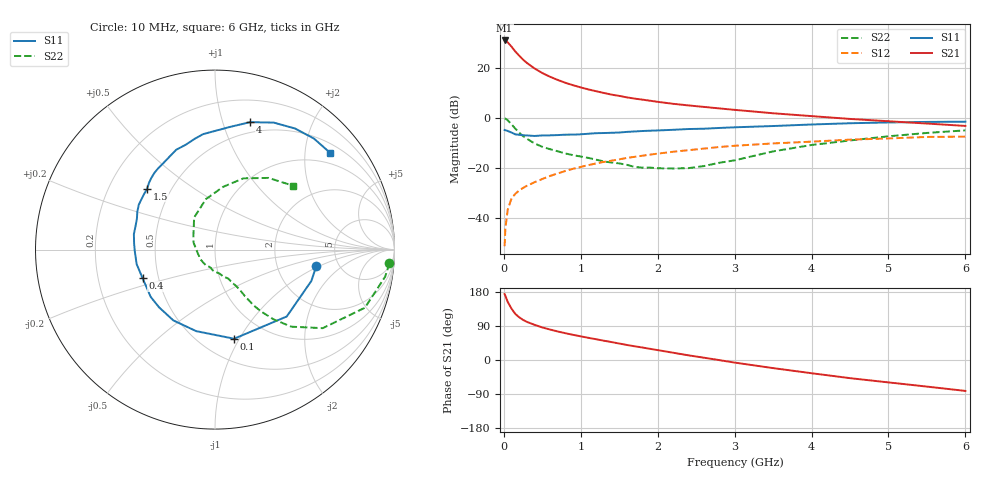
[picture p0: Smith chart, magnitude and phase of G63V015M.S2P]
! SIEMENS Small Signal Semiconductors
! BFG193
! Si NPN RF Bipolar Junction Transistor in SOT223
! VCE = 3 V  IC = 15 mA
! Common Emitter S-Parameters:  August  1996
# GHz  S  MA  R  50
!  f  S11  S21  S12  S22
! GHz  MAG  ANG  MAG  ANG  MAG  ANG  MAG  ANG
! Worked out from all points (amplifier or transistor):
!   36 points, 10 MHz to 6 GHz, reference 50 ohm
!   highest |S21| = 31.0 dB at 10 MHz (marker M1)
!   |S21| within 3 dB of that: start of sweep to 113.4 MHz
!   unconditionally stable (mu >= 1): 762.2 MHz to 2.618 GHz
!   at 250 MHz: K = 0.66, MSG = 25.7 dB, |S12| = -28.1 dB
!   at 1.4 GHz: K = 1.06, MAG = 11.7 dB, |S12| = -17.1 dB
!   at 6 GHz: K = 0.89, MSG = 2.1 dB, |S12| = -7.5 dB
!   S11 on the Smith chart (normalised r, x): 10 MHz: 3.40, -0.92; 100 MHz: 0.71, -0.95; 400 MHz: 0.41, -0.16; 1.5 GHz: 0.37, +0.34; 4 GHz: 0.40, +1.23; 6 GHz: 0.71, +2.58
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0.01  0.5717 -9.2  35.39 174.0  0.0027 90.0  0.9745 -4.5
0.02  0.5646 -18.0  35.03 169.4  0.0061 84.9  0.9602 -9.0
0.05  0.5465 -43.0  32.41 153.5  0.0144 71.2  0.8958 -21.2
0.1  0.5078 -77.9  26.63 135.4  0.0244 63.1  0.7429 -36.1
0.15  0.4662 -103.0  21.21 121.4  0.0303 56.5  0.6042 -45.3
0.2  0.4577 -120.5  17.54 112.7  0.0352 55.7  0.5068 -50.0
0.25  0.4478 -134.1  14.63 105.8  0.0395 54.7  0.4299 -53.3
0.3  0.4447 -143.7  12.55 100.6  0.0437 55.1  0.3811 -55.2
0.4  0.4338 -158.6  9.727 92.8  0.0515 55.5  0.3075 -57.3
0.5  0.4439 -169.4  7.879 85.9  0.0597 55.9  0.2632 -58.3
0.6  0.4464 -178.1  6.647 80.4  0.0685 56.7  0.2359 -59.7
0.7  0.4517 176.0  5.739 75.3  0.0772 56.3  0.2141 -61.8
0.9  0.4611 164.1  4.495 66.4  0.0956 54.9  0.1789 -65.1
1.1  0.4808 154.2  3.701 58.5  0.1133 52.9  0.1577 -72.8
1.5  0.5083 138.0  2.748 43.5  0.1477 46.5  0.1225 -92.0
2.2  0.5763 116.1  1.91 19.2  0.2095 33.0  0.097 -146.2
2.8  0.6271 100.5  1.545 -0.3  0.2606 20.2  0.1261 161.6
3.5  0.6855 83.7  1.235 -21.4  0.3076 3.5  0.2131 123.1
4  0.736 74.7  1.083 -34.9  0.3338 -6.0  0.2859 100.2
4.5  0.7796 65.2  0.951 -47.9  0.3661 -16.2  0.3527 82.6
5.5  0.8287 48.3  0.769 -70.2  0.4146 -39.8  0.4988 53.2
6  0.838 40.0  0.689 -81.6  0.4204 -53.4  0.5619 39.3
